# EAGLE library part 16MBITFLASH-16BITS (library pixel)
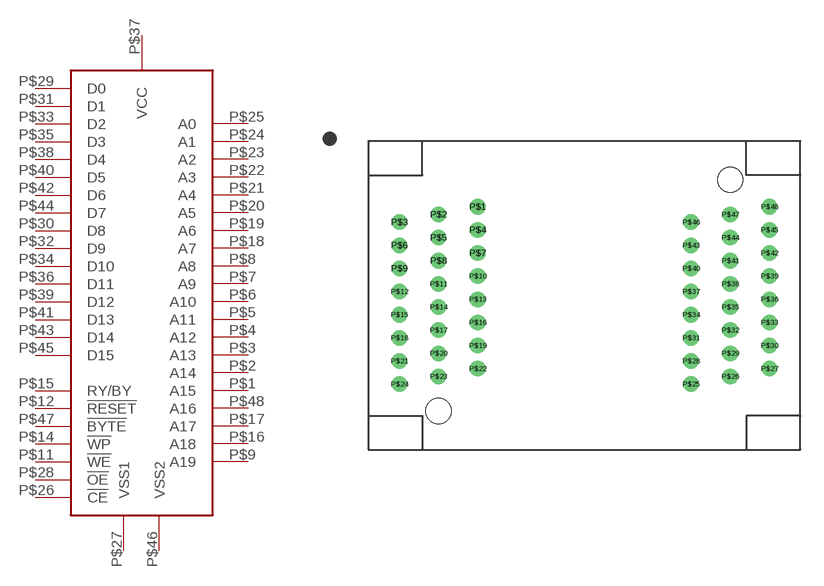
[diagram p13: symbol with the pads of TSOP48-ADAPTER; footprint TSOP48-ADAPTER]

Designator prefix -

## 16MBITFLASH-16BITS  [TSOP48-ADAPTER]
P$1  A15
P$2  A14
P$3  A13
P$4  A12
P$5  A11
P$6  A10
P$7  A9
P$8  A8
P$9  A19
P$11  !WE
P$12  !RESET
P$14  !WP
P$15  RY/BY
P$16  A18
P$17  A17
P$18  A7
P$19  A6
P$20  A5
P$21  A4
P$22  A3
P$23  A2
P$24  A1
P$25  A0
P$26  !CE
P$27  VSS1
P$28  !OE
P$29  D0
P$30  D8
P$31  D1
P$32  D9
P$33  D2
P$34  D10
P$35  D3
P$36  D11
P$37  VCC
P$38  D4
P$39  D12
P$40  D5
P$41  D13
P$42  D6
P$43  D14
P$44  D7
P$45  D15
P$46  VSS2
P$47  !BYTE
P$48  A16

## Footprint TSOP48-ADAPTER (pad centres in mm)
drill 0.5 pad 0.754: P$1 -6.915,5.75; P$2 -9.455,5.25; P$3 -11.995,4.75; P$4 -6.915,4.25; P$5 -9.455,3.75; P$6 -11.995,3.25; P$7 -6.915,2.75; P$8 -9.455,2.25; P$9 -11.995,1.75; P$10 -6.915,1.25; P$11 -9.455,0.75; P$12 -11.995,0.25; P$13 -6.915,-0.25; P$14 -9.455,-0.75; P$15 -11.995,-1.25; P$16 -6.915,-1.75; P$17 -9.455,-2.25; P$18 -11.995,-2.75; P$19 -6.915,-3.25; P$20 -9.455,-3.75; P$21 -11.995,-4.25; P$22 -6.915,-4.75; P$23 -9.455,-5.25; P$24 -11.995,-5.75; P$25 6.915,-5.75; P$26 9.455,-5.25; P$27 11.995,-4.75; P$28 6.915,-4.25; P$29 9.455,-3.75; P$30 11.995,-3.25; P$31 6.915,-2.75; P$32 9.455,-2.25; P$33 11.995,-1.75; P$34 6.915,-1.25; P$35 9.455,-0.75; P$36 11.995,-0.25; P$37 6.915,0.25; P$38 9.455,0.75; P$39 11.995,1.25; P$40 6.915,1.75; P$41 9.455,2.25; P$42 11.995,2.75; P$43 6.915,3.25; P$44 9.455,3.75; P$45 11.995,4.25; P$46 6.915,4.75; P$47 9.455,5.25; P$48 11.995,5.75
hole 1.65 at 9.455,7.5
hole 1.65 at -9.455,-7.5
